|   IBIS model for TI xxx DSP
[IBIS Ver]   5.1
[Disclaimer]   Please be aware that in the absence of a written agreement
|   Texas Instruments(TI) assumes no liability for:
|   (1) The accuracy of the IBIS models provided to your company,
|   however, the IBIS model is compliant to industry standard
|   IQ Level 2a.  Refer to IBIS Quality Section below for
|   for full details.
|   (2) The proper functioning of these Models in your design
|   or for any resulting applications
|   (3) Infringement of patents, copyrights or intellectual
|   property rights resulting from your use of these
|   models.
|   TI provides IBIS Models as a service to our customers and
|   therefore reserves the right to limit distribution of the
|   Models.  The information is subject to change without notice.
[File Name]  sprm783b.ibs
[File Rev]   0.3
|   -Removed DDR model
|   -Replaced with AM243 package models
|   -Modified pad capacitance values for LVCMOS and SDIO cells
|   -Removed untrimmed models
|   -Removed unused models for LVCMOS
[Date]   5 December 2022
[Source]   Texas Instruments Incorporated
[Copyright]   Property of Texas Instruments Incorporated.
|   Unauthorized reproduction and/or distribution is strictly.
|   prohibited.
|   This product is protected under copyright law and trade
|   secret law as an unpublished work.
|   Created 2012,(C) Copyright 1999-2012,
|   Texas Instruments Incorporated., All Rights Reserved.
|   These commodities are under the U.S. Government
|   distribution license control. As such,they are not to be
|   re-exported without the prior approval of the U.S.
|   Department of Commerce.
[Notes]
   This file does not include AMI models for SerDes based links.
   For SerDes simulations use Texas Instruments IBIS AMI models
   Some IV curves contain Non monotonic data points.
|   Revision History
|   GERNERAL COMMENT: All IBIS Quality Notes below reflect latest release
|   and version of IBIS File
|   File passes ibischk6.0 with 0 errors and 43 warnings
|   Component AM243
[Component] AM243
[Manufacturer] Texas Instruments
[Package]
|   typ   min   max
R_pkg   0.23303   0.03292   0.52144
L_pkg   1.796e-9   2.817e-10   3.851e-9
C_pkg   5.27e-13   2.202e-13   9.575e-13
[Package Model]		am243_pkg
[Pin]  Signal_name   model_name
H21	ADC0_AIN0   NC
F19	ADC0_AIN1   NC
F21	ADC0_AIN2   NC
F20	ADC0_AIN3   NC
H20	ADC0_AIN4   NC
E21	ADC0_AIN5   NC
G20	ADC0_AIN6   NC
E20	ADC0_AIN7   NC
J13	ATEST0   NC
C5	EMU0   LVCMOS_V
B3	EMU1   LVCMOS_V
A18	EXT_REFCLK1   LVCMOS_V
R21	GPMC0_AD0   LVCMOS_H
R20	GPMC0_AD1   LVCMOS_H
T19	GPMC0_AD2   LVCMOS_H
V21	GPMC0_AD3   LVCMOS_H
U21	GPMC0_AD4   LVCMOS_H
T20	GPMC0_AD5   LVCMOS_H
T18	GPMC0_AD6   LVCMOS_H
U19	GPMC0_AD7   LVCMOS_H
U18	GPMC0_AD8   LVCMOS_H
U20	GPMC0_AD9   LVCMOS_H
V20	GPMC0_AD10   LVCMOS_H
W20	GPMC0_AD11   LVCMOS_H
Y20	GPMC0_AD12   LVCMOS_H
Y19	GPMC0_AD13   LVCMOS_H
Y18	GPMC0_AD14   LVCMOS_H
AA19	GPMC0_AD15   LVCMOS_H
P21	GPMC0_BE1N   LVCMOS_H
B16	I2C0_SCL   IIC_V
B15	I2C0_SDA   IIC_V
A17	I2C1_SCL   LVCMOS_V
B18	I2C1_SDA   LVCMOS_V
A14	MCAN0_RX   LVCMOS_V
B13	MCAN0_TX   LVCMOS_V
A15	MCAN1_RX   LVCMOS_V
B14	MCAN1_TX   LVCMOS_V
D20	MCU_OSC0_XI   NC
C21	MCU_OSC0_XO   NC
C20	MCU_PORZ   RESET_H
A6	MCU_RESETSTATZ   LVCMOS_V
A5	MCU_RESETZ   LVCMOS_V
B20	MCU_SAFETY_ERRORN	LVCMOS_V
D4	MCU_UART0_CTSN   LVCMOS_V
C2	MCU_UART0_RTSN   LVCMOS_V
D6	MCU_UART0_RXD   LVCMOS_V
B2	MCU_UART0_TXD   LVCMOS_V
J20	MMC1_CLK   SDIO_H
J21	MMC1_CMD   SDIO_H
J18	MMC1_DAT0   SDIO_H
J19	MMC1_DAT1   SDIO_H
K20	MMC1_DAT2   SDIO_H
K18	MMC1_DAT3   SDIO_H
B17	MMC1_SDCD   LVCMOS_V
C16	MMC1_SDWP   LVCMOS_V
P20	OSPI0_CLK   LVCMOS_H
L20	OSPI0_CSN0   LVCMOS_H
M20	OSPI0_CSN1   LVCMOS_H
L19	OSPI0_D0   LVCMOS_H
N20	OSPI0_D1   LVCMOS_H
L21	OSPI0_D2   LVCMOS_H
N19	OSPI0_D3   LVCMOS_H
P17	OSPI0_DQS   LVCMOS_H
M21	OSPI0_LBCLKO   LVCMOS_H
D18	PORZ_OUT   LVCMOS_H
D2	PRG0_MDIO0_MDC   LVCMOS_H
E4	PRG0_MDIO0_MDIO   LVCMOS_H
J3	PRG0_PRU0_GPO0   LVCMOS_H
J4	PRG0_PRU0_GPO1   LVCMOS_H
G1	PRG0_PRU0_GPO2   LVCMOS_H
H1	PRG0_PRU0_GPO3   LVCMOS_H
K2	PRG0_PRU0_GPO4   LVCMOS_H
F2	PRG0_PRU0_GPO5   LVCMOS_H
H2	PRG0_PRU0_GPO6   LVCMOS_H
E2	PRG0_PRU0_GPO7   LVCMOS_H
H5	PRG0_PRU0_GPO8   LVCMOS_H
Y3	PRG0_PRU0_GPO9   LVCMOS_H
U1	PRG0_PRU0_GPO10   LVCMOS_H
L1	PRG0_PRU0_GPO11   LVCMOS_H
K1	PRG0_PRU0_GPO12   LVCMOS_H
N1	PRG0_PRU0_GPO13   LVCMOS_H
N2	PRG0_PRU0_GPO14   LVCMOS_H
N4	PRG0_PRU0_GPO15   LVCMOS_H
N3	PRG0_PRU0_GPO16   LVCMOS_H
E1	PRG0_PRU0_GPO17   LVCMOS_H
K4	PRG0_PRU0_GPO18   LVCMOS_H
G2	PRG0_PRU0_GPO19   LVCMOS_H
L5	PRG0_PRU1_GPO0   LVCMOS_H
J2	PRG0_PRU1_GPO1   LVCMOS_H
M2	PRG0_PRU1_GPO2   LVCMOS_H
L2	PRG0_PRU1_GPO3   LVCMOS_H
L3	PRG0_PRU1_GPO4   LVCMOS_H
E3	PRG0_PRU1_GPO5   LVCMOS_H
F5	PRG0_PRU1_GPO6   LVCMOS_H
T5	PRG0_PRU1_GPO7   LVCMOS_H
F4	PRG0_PRU1_GPO8   LVCMOS_H
R2	PRG0_PRU1_GPO9   LVCMOS_H
U2	PRG0_PRU1_GPO10   LVCMOS_H
P1	PRG0_PRU1_GPO11   LVCMOS_H
P2	PRG0_PRU1_GPO12   LVCMOS_H
T4	PRG0_PRU1_GPO13   LVCMOS_H
R5	PRG0_PRU1_GPO14   LVCMOS_H
M4	PRG0_PRU1_GPO15   LVCMOS_H
T3	PRG0_PRU1_GPO16   LVCMOS_H
T1	PRG0_PRU1_GPO17   LVCMOS_H
D1	PRG0_PRU1_GPO18   LVCMOS_H
F3	PRG0_PRU1_GPO19   LVCMOS_H
W1	PRG1_MDIO0_MDC   LVCMOS_V
V2	PRG1_MDIO0_MDIO   LVCMOS_V
V4	PRG1_PRU0_GPO0   LVCMOS_V
W5	PRG1_PRU0_GPO1   LVCMOS_V
AA4	PRG1_PRU0_GPO2   LVCMOS_V
Y5	PRG1_PRU0_GPO3   LVCMOS_V
AA5	PRG1_PRU0_GPO4   LVCMOS_V
U14	PRG1_PRU0_GPO5   LVCMOS_V
Y2	PRG1_PRU0_GPO6   LVCMOS_V
V13	PRG1_PRU0_GPO7   LVCMOS_V
Y13	PRG1_PRU0_GPO8   LVCMOS_V
W16	PRG1_PRU0_GPO9   LVCMOS_V
W13	PRG1_PRU0_GPO10   LVCMOS_V
V5	PRG1_PRU0_GPO11   LVCMOS_V
W2	PRG1_PRU0_GPO12   LVCMOS_V
V6	PRG1_PRU0_GPO13   LVCMOS_V
AA7	PRG1_PRU0_GPO14   LVCMOS_V
Y7	PRG1_PRU0_GPO15   LVCMOS_V
W6	PRG1_PRU0_GPO16   LVCMOS_V
T2	PRG1_PRU0_GPO17   LVCMOS_V
Y4	PRG1_PRU0_GPO18   LVCMOS_V
U3	PRG1_PRU0_GPO19   LVCMOS_V
AA10	PRG1_PRU1_GPO0   LVCMOS_V
Y10	PRG1_PRU1_GPO1   LVCMOS_V
Y11	PRG1_PRU1_GPO2   LVCMOS_V
V12	PRG1_PRU1_GPO3   LVCMOS_V
Y12	PRG1_PRU1_GPO4   LVCMOS_V
AA11	PRG1_PRU1_GPO5   LVCMOS_V
V10	PRG1_PRU1_GPO6   LVCMOS_V
Y14	PRG1_PRU1_GPO7   LVCMOS_V
W11	PRG1_PRU1_GPO8   LVCMOS_V
Y16	PRG1_PRU1_GPO9   LVCMOS_V
U13	PRG1_PRU1_GPO10   LVCMOS_V
Y6	PRG1_PRU1_GPO11   LVCMOS_V
AA8	PRG1_PRU1_GPO12   LVCMOS_V
Y9	PRG1_PRU1_GPO13   LVCMOS_V
W9	PRG1_PRU1_GPO14   LVCMOS_V
V9	PRG1_PRU1_GPO15   LVCMOS_V
Y8	PRG1_PRU1_GPO16   LVCMOS_V
AA14	PRG1_PRU1_GPO17   LVCMOS_V
Y15	PRG1_PRU1_GPO18   LVCMOS_V
AA13	PRG1_PRU1_GPO19   LVCMOS_V
E19	RESETSTATZ   LVCMOS_V
C17	RESET_REQZ   LVCMOS_V
B8	SPI0_CLK   LVCMOS_V
B7	SPI0_CS1   LVCMOS_V
A8	SPI0_D0   LVCMOS_V
C9	SPI0_D1   LVCMOS_V
C6	TCK   LVCMOS_V
A3	TDI   LVCMOS_V
B5	TDO   LVCMOS_V
H11	TEMP_DIODE_P   NC
B4	TMS   LVCMOS_V
B6	TRSTN   LVCMOS_V
B9	UART0_CTSN   LVCMOS_V
A9	UART0_RTSN   LVCMOS_V
B10	UART0_RXD   LVCMOS_V
B11	UART0_TXD   LVCMOS_V
C11	UART1_CTSN   LVCMOS_V
A11	UART1_RTSN   LVCMOS_V
B12	UART1_RXD   LVCMOS_V
A12	UART1_TXD   LVCMOS_V
AA17	USB0_DM   NC
AA16	USB0_DP   NC
B19	USB0_DRVVBUS   LVCMOS_V
Y17	USB0_ID   NC
W17	USB0_RCALIB   NC
V18	USB0_VBUS   NC
F14	VMON_1P8_SOC   POWER
E15	VMON_3P3_SOC   POWER
G13	VMON_VSYS   POWER
A21   VSS   GND
B21   VSS   GND
A20   VSS   GND
A2   VSS   GND
A1   VSS   GND
B1   VSS   GND
D17   VSS   GND
D16   VSS   GND
E11   VSS   GND
D10   VSS   GND
E6   VSS   GND
F17   VSS   GND
F8   VSS   GND
G16   VSS   GND
H16   VSS   GND
H7   VSS   GND
H6   VSS   GND
J16   VSS   GND
J11   VSS   GND
J5   VSS   GND
J6   VSS   GND
K16   VSS   GND
L11   VSS   GND
L12   VSS   GND
L10   VSS   GND
K8   VSS   GND
K7   VSS   GND
K6   VSS   GND
M16   VSS   GND
M15   VSS   GND
M7   VSS   GND
P16   VSS   GND
P15   VSS   GND
N13   VSS   GND
N11   VSS   GND
P11   VSS   GND
P7   VSS   GND
N6   VSS   GND
R11   VSS   GND
R6   VSS   GND
T14   VSS   GND
U6   VSS   GND
Y21   VSS   GND
Y1   VSS   GND
AA21   VSS   GND
AA20   VSS   GND
AA2   VSS   GND
AA1   VSS   GND
E13   VSS   GND
D12   CAP_VDDS0   POWER
N5   CAP_VDDS1   POWER
U9   CAP_VDDS2   POWER
R16   CAP_VDDS3   POWER
N18   CAP_VDDS4   POWER
M18   CAP_VDDS5   POWER
J17   CAP_VDDSHV_MMC1   POWER
D9   CAP_VDDS_MCU   POWER
V16   VDDA_0P85_USB0   POWER
U15   VDDA_1P8_USB0   POWER
K15   VDDA_3P3_SDIO   POWER
U16   VDDA_3P3_USB0   POWER
H17   VDDA_ADC   POWER
G17   VDDA_ADC   POWER
H14   VDDA_MCU   POWER
N12   VDDA_PLL0   POWER
G9   VDDA_PLL1   POWER
G12   VDDA_PLL2   POWER
G11   VDDA_TEMP0   POWER
M11   VDDA_TEMP1   POWER
P14   VDDR_CORE   POWER
J12   VDDR_CORE   POWER
J10   VDDR_CORE   POWER
R10   VDDR_CORE   POWER
P8   VDDR_CORE   POWER
G6   VDDR_CORE   POWER
G5   VDDR_CORE   POWER
E14   VDDSHV0   POWER
D13   VDDSHV0   POWER
C13   VDDSHV0   POWER
L6   VDDSHV1   POWER
M6   VDDSHV1   POWER
P5   VDDSHV1   POWER
P6   VDDSHV1   POWER
T11   VDDSHV2   POWER
U11   VDDSHV2   POWER
T8   VDDSHV2   POWER
U8   VDDSHV2   POWER
U7   VDDSHV2   POWER
R17   VDDSHV3   POWER
T17   VDDSHV3   POWER
N17   VDDSHV4   POWER
N16   VDDSHV4   POWER
L17   VDDSHV5   POWER
L16   VDDSHV5   POWER
E8   VDDSHV_MCU   POWER
E9   VDDSHV_MCU   POWER
E7   VDDSHV_MCU   POWER
F18   VDDS_OSC   POWER
H15   VDD_CORE   POWER
K14   VDD_CORE   POWER
L13   VDD_CORE   POWER
M14   VDD_CORE   POWER
R13   VDD_CORE   POWER
R12   VDD_CORE   POWER
K11   VDD_CORE   POWER
G10   VDD_CORE   POWER
N10   VDD_CORE   POWER
N9   VDD_CORE   POWER
H8   VDD_CORE   POWER
J9   VDD_CORE   POWER
L9   VDD_CORE   POWER
M8   VDD_CORE   POWER
R9   VDD_CORE   POWER
F11   VDD_CORE   POWER
E16   VPP   POWER
|****************** SDIO
[Model Selector] SDIO_H
sdio1_r33_1p8_h PRWDWUWSWEWCDGSDIO_H@_R33_1p8_comment
sdio1_r33_3p3_h PRWDWUWSWEWCDGSDIO_H@_R33_3p3_comment
sdio1_r40_1p8_h PRWDWUWSWEWCDGSDIO_H@_R40_1p8_comment
sdio1_r40_3p3_h PRWDWUWSWEWCDGSDIO_H@_R40_3p3_comment
sdio1_r50_1p8_h PRWDWUWSWEWCDGSDIO_H@_R50_1p8_comment
sdio1_r50_3p3_h PRWDWUWSWEWCDGSDIO_H@_R50_3p3_comment
sdio1_r66_1p8_h PRWDWUWSWEWCDGSDIO_H@_R66_1p8_comment
sdio1_r66_3p3_h PRWDWUWSWEWCDGSDIO_H@_R66_3p3_comment
|********** LVCMOS
[Model Selector] LVCMOS_H
lvcmos1_nom_1p8_h PRWDWUWSWEWCDGLVCMOS_H@_Nom_1p8_comment
lvcmos1_nom_3p3_h PRWDWUWSWEWCDGLVCMOS_H@_Nom_3p3_comment
[Model Selector] LVCMOS_V
lvcmos0_nom_1p8_v PRWDWUWSWEWCDGLVCMOS_V@_Nom_1p8_comment
lvcmos0_nom_3p3_v PRWDWUWSWEWCDGLVCMOS_V@_Nom_3p3_comment
[Model Selector] IIC_V
IIC18_1_0_V PRBOPDDGZIIC_V@HSMODE_HSMCSE=0_0_comment 1.8V
IIC18_1_1_V PRBOPDDGZIIC_V@HSMODE_HSMCSE=0_1_comment 1.8V
IIC18_1_2_V PRBOPDDGZIIC_V@HSMODE_HSMCSE=1_0_comment 1.8V
IIC18_1_3_V PRBOPDDGZIIC_V@HSMODE_HSMCSE=1_1_comment 1.8V
IIC33_1_0_V PRBOPDDGZIIC_V@HSMODE_HSMCSE=0_0_comment
IIC33_1_1_V PRBOPDDGZIIC_V@HSMODE_HSMCSE=0_1_comment
IIC33_1_2_V PRBOPDDGZIIC_V@HSMODE_HSMCSE=1_0_comment
IIC33_1_3_V PRBOPDDGZIIC_V@HSMODE_HSMCSE=1_1_comment
|***************** RESET ************************************************
[Model Selector] RESET_H
reset18_0_0 PDIDGZRESET_H
|   EMMC
[MODEL SELECTOR] EMMC
emmc51_io_tx33ohm   33ohm DRIVER
emmc51_io_tx40ohm   40ohm DRIVER
emmc51_io_tx50ohm   50ohm DRIVER
emmc51_io_tx66ohm   66ohm DRIVER
emmc51_io_tx100ohm  100ohm DRIVER
emmc51_io_txod   Open drain DRIVER
|   Package Model
[Define Package Model]   am243_pkg
[Manufacturer]   name 1
[OEM]   name 2
[Description]   208-pin Package
|[Number of Sections]   1
[Number of Pins]   208
[Pin Numbers]
|[Pin Name]  Net Number   Net Name   Net's All Pins
D12   | 1   CAP_VDDS0   D12
N5   | 2   CAP_VDDS1   N5
U9   | 3   CAP_VDDS2   U9
R16   | 4   CAP_VDDS3   R16
N18   | 5   CAP_VDDS4   N18
M18   | 6   CAP_VDDS5   M18
J17   | 7   CAP_VDDSHV_MMC1   J17
D9   | 8   CAP_VDDS_MCU   D9
V16   | 9   VDDA_0P85_USB0   V16
U15   | 10   VDDA_1P8_USB0   U15
K15   | 11   VDDA_3P3_SDIO   K15
U16   | 12   VDDA_3P3_USB0   U16
H17   | 13   VDDA_ADC   H17
   |G17
H14   | 14   VDDA_MCU   H14
N12   | 15   VDDA_PLL0   N12
G9   | 16   VDDA_PLL1   G9
G12   | 17   VDDA_PLL2   G12
G11   | 18   VDDA_TEMP0   G11
M11   | 19   VDDA_TEMP1   M11
P14   | 20   VDDR_CORE   P14
   |J12
   |J10
   |R10
   |P8
   |G6
   |G5
E14   | 21   VDDSHV0   E14
   |D13
   |C13
L6   | 22   VDDSHV1   L6
   |M6
   |P5
   |P6
T11   | 23   VDDSHV2   T11
   |U11
   |T8
   |U8
   |U7
R17   | 24   VDDSHV3   R17
   |T17
N17   | 25   VDDSHV4   N17
   |N16
L17   | 26   VDDSHV5   L17
   |L16
E8   | 27   VDDSHV_MCU   E8
   |E9
   |E7
F18   | 28   VDDS_OSC   F18
H15   | 29   VDD_CORE   H15
   |K14
   |L13
   |M14
   |R13
   |R12
   |K11
   |G10
   |N10
   |N9
   |H8
   |J9
   |L9
   |M8
   |R9
   |F11
E16   | 30   VPP   E16
H21   | 31   ADC0_AIN0   H21
F19   | 32   ADC0_AIN1   F19
F21   | 33   ADC0_AIN2   F21
F20   | 34   ADC0_AIN3   F20
H20   | 35   ADC0_AIN4   H20
E21   | 36   ADC0_AIN5   E21
G20   | 37   ADC0_AIN6   G20
E20   | 38   ADC0_AIN7   E20
J13   | 39   ATEST0   J13
C5   | 40   EMU0   C5
B3   | 41   EMU1   B3
A18   | 42   EXT_REFCLK1   A18
R21   | 43   GPMC0_AD0   R21
R20   | 44   GPMC0_AD1   R20
T19   | 45   GPMC0_AD2   T19
V21   | 46   GPMC0_AD3   V21
U21   | 47   GPMC0_AD4   U21
T20   | 48   GPMC0_AD5   T20
T18   | 49   GPMC0_AD6   T18
U19   | 50   GPMC0_AD7   U19
U18   | 51   GPMC0_AD8   U18
U20   | 52   GPMC0_AD9   U20
V20   | 53   GPMC0_AD10   V20
W20   | 54   GPMC0_AD11   W20
Y20   | 55   GPMC0_AD12   Y20
Y19   | 56   GPMC0_AD13   Y19
Y18   | 57   GPMC0_AD14   Y18
AA19   | 58   GPMC0_AD15   AA19
P21   | 59   GPMC0_BE1N   P21
B16   | 60   I2C0_SCL   B16
B15   | 61   I2C0_SDA   B15
A17   | 62   I2C1_SCL   A17
B18   | 63   I2C1_SDA   B18
A14   | 64   MCAN0_RX   A14
B13   | 65   MCAN0_TX   B13
A15   | 66   MCAN1_RX   A15
B14   | 67   MCAN1_TX   B14
D20   | 68   MCU_OSC0_XI   D20
C21   | 69   MCU_OSC0_XO   C21
C20   | 70   MCU_PORZ   C20
A6   | 71   MCU_RESETSTATZ   A6
A5   | 72   MCU_RESETZ   A5
B20   | 73   MCU_SAFETY_ERRORN   B20
D4   | 74   MCU_UART0_CTSN   D4
C2   | 75   MCU_UART0_RTSN   C2
D6   | 76   MCU_UART0_RXD   D6
B2   | 77   MCU_UART0_TXD   B2
J20   | 78   MMC1_CLK   J20
J21   | 79   MMC1_CMD   J21
J18   | 80   MMC1_DAT0   J18
J19   | 81   MMC1_DAT1   J19
K20   | 82   MMC1_DAT2   K20
K18   | 83   MMC1_DAT3   K18
B17   | 84   MMC1_SDCD   B17
C16   | 85   MMC1_SDWP   C16
P20   | 86   OSPI0_CLK   P20
L20   | 87   OSPI0_CSN0   L20
M20   | 88   OSPI0_CSN1   M20
L19   | 89   OSPI0_D0   L19
N20   | 90   OSPI0_D1   N20
L21   | 91   OSPI0_D2   L21
N19   | 92   OSPI0_D3   N19
P17   | 93   OSPI0_DQS   P17
M21   | 94   OSPI0_LBCLKO   M21
D18   | 95   PORZ_OUT   D18
D2   | 96   PRG0_MDIO0_MDC   D2
E4   | 97   PRG0_MDIO0_MDIO   E4
J3   | 98   PRG0_PRU0_GPO0   J3
J4   | 99   PRG0_PRU0_GPO1   J4
G1   | 100   PRG0_PRU0_GPO2   G1
H1   | 101   PRG0_PRU0_GPO3   H1
K2   | 102   PRG0_PRU0_GPO4   K2
F2   | 103   PRG0_PRU0_GPO5   F2
H2   | 104   PRG0_PRU0_GPO6   H2
E2   | 105   PRG0_PRU0_GPO7   E2
H5   | 106   PRG0_PRU0_GPO8   H5
Y3   | 107   PRG0_PRU0_GPO9   Y3
U1   | 108   PRG0_PRU0_GPO10   U1
L1   | 109   PRG0_PRU0_GPO11   L1
K1   | 110   PRG0_PRU0_GPO12   K1
N1   | 111   PRG0_PRU0_GPO13   N1
N2   | 112   PRG0_PRU0_GPO14   N2
N4   | 113   PRG0_PRU0_GPO15   N4
N3   | 114   PRG0_PRU0_GPO16   N3
E1   | 115   PRG0_PRU0_GPO17   E1
K4   | 116   PRG0_PRU0_GPO18   K4
G2   | 117   PRG0_PRU0_GPO19   G2
L5   | 118   PRG0_PRU1_GPO0   L5
J2   | 119   PRG0_PRU1_GPO1   J2
M2   | 120   PRG0_PRU1_GPO2   M2
L2   | 121   PRG0_PRU1_GPO3   L2
L3   | 122   PRG0_PRU1_GPO4   L3
E3   | 123   PRG0_PRU1_GPO5   E3
F5   | 124   PRG0_PRU1_GPO6   F5
T5   | 125   PRG0_PRU1_GPO7   T5
F4   | 126   PRG0_PRU1_GPO8   F4
R2   | 127   PRG0_PRU1_GPO9   R2
U2   | 128   PRG0_PRU1_GPO10   U2
P1   | 129   PRG0_PRU1_GPO11   P1
P2   | 130   PRG0_PRU1_GPO12   P2
T4   | 131   PRG0_PRU1_GPO13   T4
R5   | 132   PRG0_PRU1_GPO14   R5
M4   | 133   PRG0_PRU1_GPO15   M4
T3   | 134   PRG0_PRU1_GPO16   T3
T1   | 135   PRG0_PRU1_GPO17   T1
D1   | 136   PRG0_PRU1_GPO18   D1
F3   | 137   PRG0_PRU1_GPO19   F3
W1   | 138   PRG1_MDIO0_MDC   W1
V2   | 139   PRG1_MDIO0_MDIO   V2
V4   | 140   PRG1_PRU0_GPO0   V4
W5   | 141   PRG1_PRU0_GPO1   W5
AA4   | 142   PRG1_PRU0_GPO2   AA4
Y5   | 143   PRG1_PRU0_GPO3   Y5
AA5   | 144   PRG1_PRU0_GPO4   AA5
U14   | 145   PRG1_PRU0_GPO5   U14
Y2   | 146   PRG1_PRU0_GPO6   Y2
V13   | 147   PRG1_PRU0_GPO7   V13
Y13   | 148   PRG1_PRU0_GPO8   Y13
W16   | 149   PRG1_PRU0_GPO9   W16
W13   | 150   PRG1_PRU0_GPO10   W13
V5   | 151   PRG1_PRU0_GPO11   V5
W2   | 152   PRG1_PRU0_GPO12   W2
V6   | 153   PRG1_PRU0_GPO13   V6
AA7   | 154   PRG1_PRU0_GPO14   AA7
Y7   | 155   PRG1_PRU0_GPO15   Y7
W6   | 156   PRG1_PRU0_GPO16   W6
T2   | 157   PRG1_PRU0_GPO17   T2
Y4   | 158   PRG1_PRU0_GPO18   Y4
U3   | 159   PRG1_PRU0_GPO19   U3
AA10   | 160   PRG1_PRU1_GPO0   AA10
Y10   | 161   PRG1_PRU1_GPO1   Y10
Y11   | 162   PRG1_PRU1_GPO2   Y11
V12   | 163   PRG1_PRU1_GPO3   V12
Y12   | 164   PRG1_PRU1_GPO4   Y12
AA11   | 165   PRG1_PRU1_GPO5   AA11
V10   | 166   PRG1_PRU1_GPO6   V10
Y14   | 167   PRG1_PRU1_GPO7   Y14
W11   | 168   PRG1_PRU1_GPO8   W11
Y16   | 169   PRG1_PRU1_GPO9   Y16
U13   | 170   PRG1_PRU1_GPO10   U13
Y6   | 171   PRG1_PRU1_GPO11   Y6
AA8   | 172   PRG1_PRU1_GPO12   AA8
Y9   | 173   PRG1_PRU1_GPO13   Y9
W9   | 174   PRG1_PRU1_GPO14   W9
V9   | 175   PRG1_PRU1_GPO15   V9
Y8   | 176   PRG1_PRU1_GPO16   Y8
AA14   | 177   PRG1_PRU1_GPO17   AA14
Y15   | 178   PRG1_PRU1_GPO18   Y15
AA13   | 179   PRG1_PRU1_GPO19   AA13
E19   | 180   RESETSTATZ   E19
C17   | 181   RESET_REQZ   C17
B8   | 182   SPI0_CLK   B8
B7   | 183   SPI0_CS1   B7
A8   | 184   SPI0_D0   A8
C9   | 185   SPI0_D1   C9
C6   | 186   TCK   C6
A3   | 187   TDI   A3
B5   | 188   TDO   B5
H11   | 189   TEMP_DIODE_P   H11
B4   | 190   TMS   B4
B6   | 191   TRSTN   B6
B9   | 192   UART0_CTSN   B9
A9   | 193   UART0_RTSN   A9
B10   | 194   UART0_RXD   B10
B11   | 195   UART0_TXD   B11
C11   | 196   UART1_CTSN   C11
A11   | 197   UART1_RTSN   A11
B12   | 198   UART1_RXD   B12
A12   | 199   UART1_TXD   A12
AA17   | 200   USB0_DM   AA17
AA16   | 201   USB0_DP   AA16
B19   | 202   USB0_DRVVBUS   B19
Y17   | 203   USB0_ID   Y17
W17   | 204   USB0_RCALIB   W17
V18   | 205   USB0_VBUS   V18
F14   | 206   VMON_1P8_SOC   F14
E15   | 207   VMON_3P3_SOC   E15
G13   | 208   VMON_VSYS   G13
[Model Data]
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[End Model Data]
[End Package Model]
| Models and submodels in the file (27): lvcmos1_nom_1p8_h (I/O), lvcmos0_nom_1p8_v (I/O), lvcmos1_nom_3p3_h (I/O), lvcmos0_nom_3p3_v (I/O), sdio1_r33_1p8_h (I/O), sdio1_r33_3p3_h (I/O), sdio1_r40_1p8_h (I/O), sdio1_r40_3p3_h (I/O), sdio1_r50_1p8_h (I/O), sdio1_r50_3p3_h (I/O), sdio1_r66_1p8_h (I/O), sdio1_r66_3p3_h (I/O), emmc51_io_tx33ohm (I/O), emmc51_io_tx40ohm (I/O), emmc51_io_tx50ohm (I/O), emmc51_io_tx66ohm (I/O), emmc51_io_tx100ohm (I/O), emmc51_io_txod (I/O_open_drain), IIC33_1_0_V (I/O_open_drain), IIC33_1_1_V (I/O_open_drain), IIC33_1_2_V (I/O_open_drain), IIC33_1_3_V (I/O_open_drain), IIC18_1_0_V (I/O_open_drain), IIC18_1_1_V (I/O_open_drain), IIC18_1_2_V (I/O_open_drain), IIC18_1_3_V (I/O_open_drain), reset18_0_0 (Input)
